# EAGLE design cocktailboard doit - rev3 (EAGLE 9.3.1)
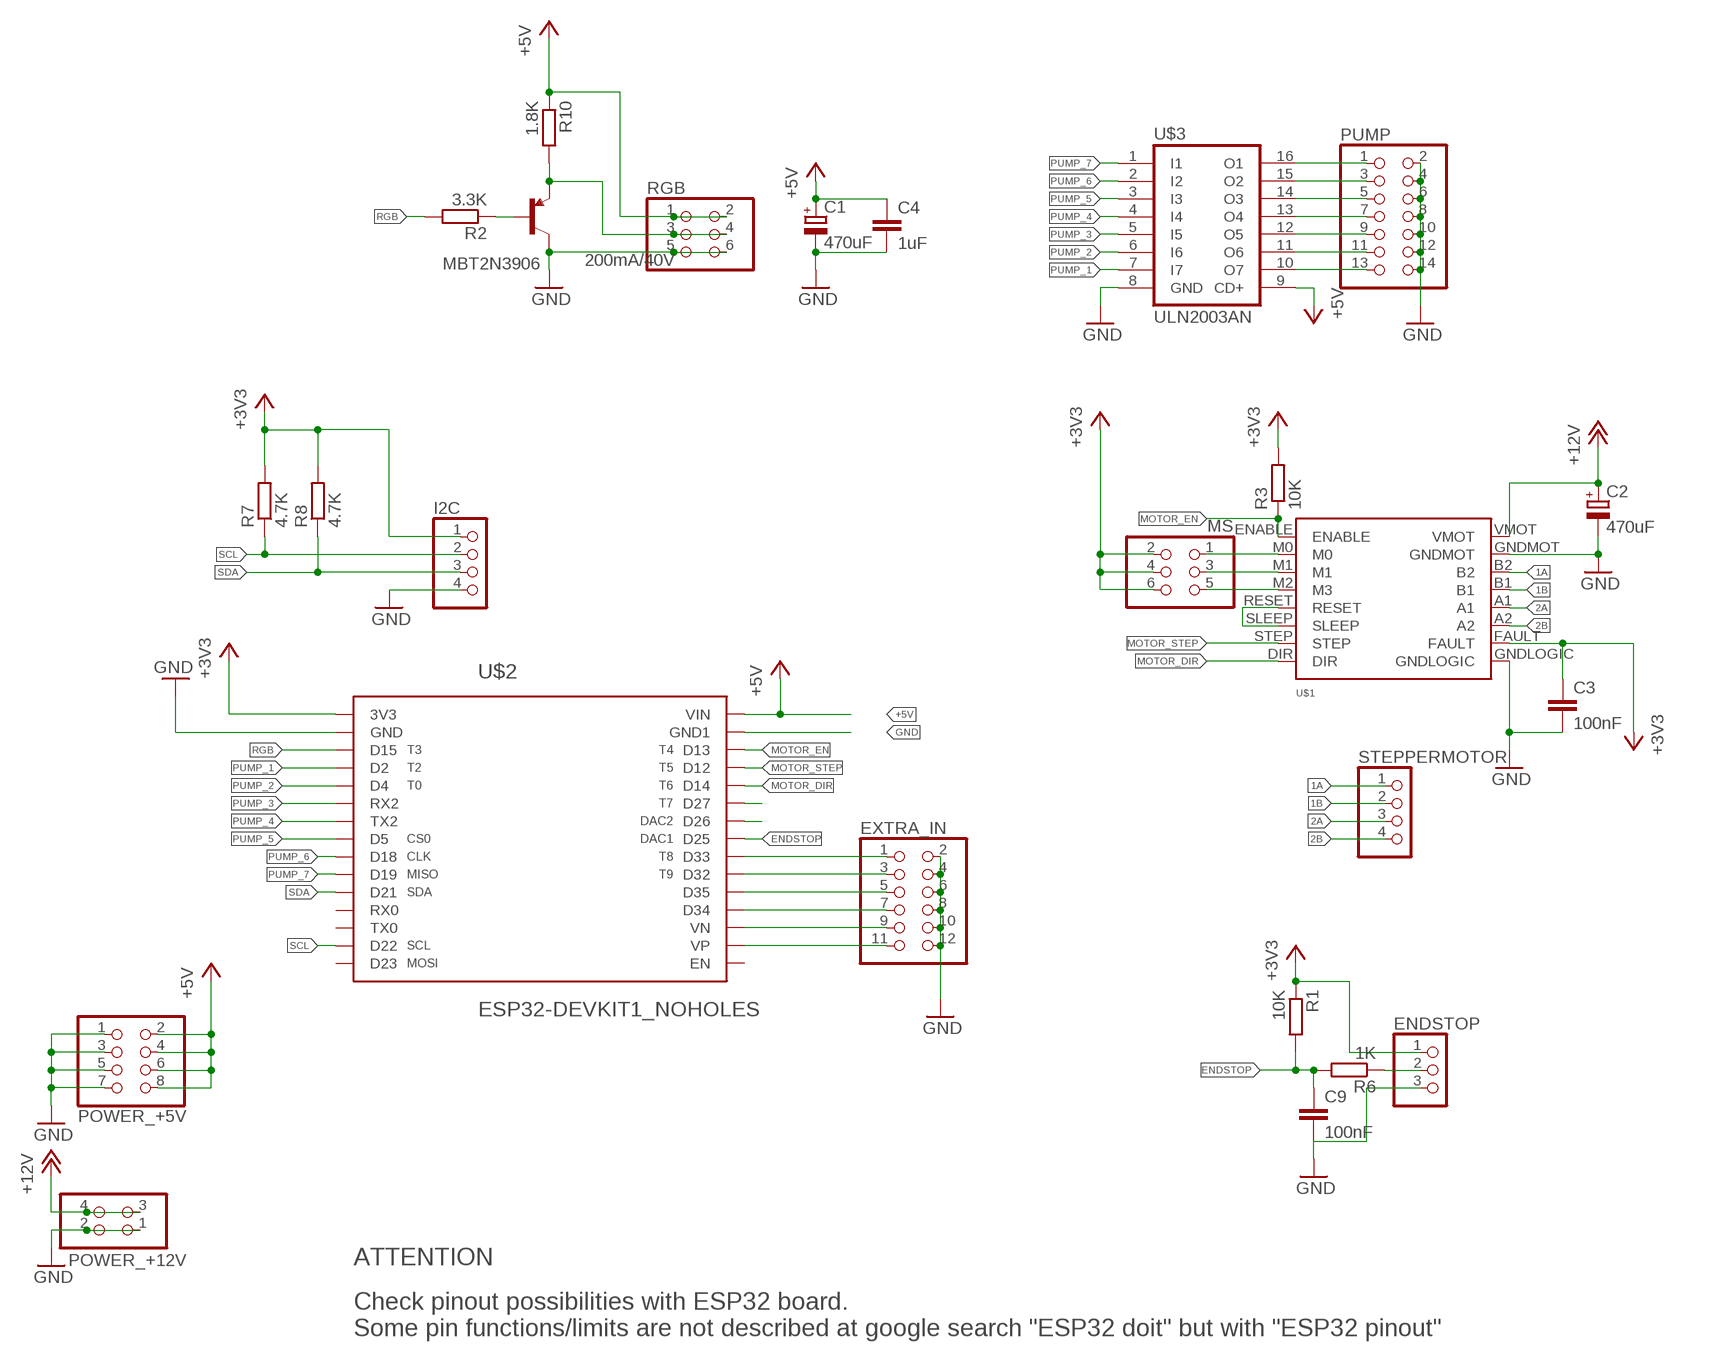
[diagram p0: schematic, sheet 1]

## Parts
C1  470uF  CPOL-EUE3.5-8  [E3,5-8]
C2  470uF  CPOL-EUE3.5-8  [E3,5-8]
C3  100nF  C-EUC1206  [C1206]
C4  1uF  C-EUC1206  [C1206]
C9  100nF  C-EUC1206  [C1206]
ENDSTOP  PINHD-1X3  [1X03]
EXTRA_IN  PINHD-2X6  [2X06]
I2C  PINHD-1X4  [1X04]
MBT2N3906  200mA/40V  TRANS_PNP-PMBT3906|MMBT3906L  [SOT23-3]
MS  PINHD-2X3  [2X03]
POWER_+5V  PINHD-2X4  [2X04]
POWER_+12V  PINHD-2X2  [2X02]
PUMP  PINHD-2X7  [2X07]
R1  10K  R-EU_R1206  [R1206]
R2  3.3K  R-EU_R1206  [R1206]
R3  10K  R-EU_R1206  [R1206]
R6  1K  R-EU_R1206  [R1206]
R7  4.7K  R-EU_R1206  [R1206]
R8  4.7K  R-EU_R1206  [R1206]
R10  1.8K  R-EU_R1206  [R1206]
RGB  PINHD-2X3  [2X03]
STEPPERMOTOR  PINHD-1X4  [1X04]
U$1  DRV8825  [DRV8825]
U$2  ESP32-DEVKIT1_NOHOLES  [NODELUA-ESP32DEVKIT1-NOHOLES]
U$3  ULN2003AN  [DIL16]

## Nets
1A: STEPPERMOTOR.1 U$1.B2
1B: STEPPERMOTOR.2 U$1.B1
2A: STEPPERMOTOR.3 U$1.A1
2B: STEPPERMOTOR.4 U$1.A2
+3V3: C3.1 ENDSTOP.1 I2C.1 MS.2 MS.4 MS.6 R1.1 R3.2 R7.2 R8.2 U$1.FAULT U$2.P$1(3V3)
+5V: C1.+ C4.1 POWER_+5V.2 POWER_+5V.4 POWER_+5V.6 POWER_+5V.8 R10.1 RGB.1 RGB.2 U$2.P$30(VIN) U$3.9(CD+)
+12V: C2.+ POWER_+12V.3 POWER_+12V.4 U$1.VMOT
ENDSTOP: C9.1 R1.2 R6.2 U$2.P$23(D25)
GND: C1.- C2.- C3.2 C4.2 C9.2 ENDSTOP.3 EXTRA_IN.2 EXTRA_IN.4 EXTRA_IN.6 EXTRA_IN.8 EXTRA_IN.10 EXTRA_IN.12 I2C.4 MBT2N3906.3(C) POWER_+5V.1 POWER_+5V.3 POWER_+5V.5 POWER_+5V.7 POWER_+12V.1 POWER_+12V.2 PUMP.2 PUMP.4 PUMP.6 PUMP.8 PUMP.10 PUMP.12 PUMP.14 RGB.5 RGB.6 U$1.GNDLOGIC U$1.GNDMOT U$2.P$2(GND) U$2.P$29(GND1) U$3.8(GND)
MOTOR_DIR: U$1.DIR U$2.P$26(D14)
MOTOR_EN: R3.1 U$1.ENABLE U$2.P$28(D13)
MOTOR_STEP: U$1.STEP U$2.P$27(D12)
N$1: MBT2N3906.1(B) R2.1
N$2: MS.1 U$1.M0
N$3: MS.3 U$1.M1
N$4: MS.5 U$1.M2(M3)
N$5: U$1.RESET U$1.SLEEP
N$6: ENDSTOP.2 R6.1
N$7: MBT2N3906.2(E) R10.2 RGB.3 RGB.4
N$8: PUMP.1 U$3.16(O1)
N$9: PUMP.3 U$3.15(O2)
N$10: PUMP.5 U$3.14(O3)
N$11: PUMP.7 U$3.13(O4)
N$12: PUMP.9 U$3.12(O5)
N$13: PUMP.11 U$3.11(O6)
N$14: PUMP.13 U$3.10(O7)
N$15: EXTRA_IN.1 U$2.P$22(D33)
N$16: EXTRA_IN.3 U$2.P$21(D32)
N$17: EXTRA_IN.5 U$2.P$20(D35)
N$18: U$2.P$25(D27)
N$19: U$2.P$24(D26)
N$20: EXTRA_IN.7 U$2.P$19(D34)
N$21: EXTRA_IN.9 U$2.P$18(VN)
N$22: EXTRA_IN.11 U$2.P$17(VP)
PUMP_1: U$2.P$4(D2) U$3.7(I7)
PUMP_2: U$2.P$5(D4) U$3.6(I6)
PUMP_3: U$2.P$6(RX2) U$3.5(I5)
PUMP_4: U$2.P$7(TX2) U$3.4(I4)
PUMP_5: U$2.P$8(D5) U$3.3(I3)
PUMP_6: U$2.P$9(D18) U$3.2(I2)
PUMP_7: U$2.P$10(D19) U$3.1(I1)
RGB: R2.2 U$2.P$3(D15)
SCL: I2C.2 R7.1 U$2.P$14(D22)
SDA: I2C.3 R8.1 U$2.P$11(D21)
Unconnected: U$2.P$12(RX0) U$2.P$13(TX0) U$2.P$15(D23) U$2.P$16(EN)

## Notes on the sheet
- ATTENTION
- Check pinout possibilities with ESP32 board.
  Some pin functions/limits are not described at google search "ESP32 doit" but with "ESP32 pinout"

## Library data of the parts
C1 C2 = resistor:CPOL-EU: POLARIZED CAPACITOR, European symbol
C3 C4 C9 = resistor:C-EU: CAPACITOR, European symbol
ENDSTOP = pinhead:PINHD-1X3: PIN HEADER
EXTRA_IN = pinhead:PINHD-2X6: PIN HEADER
I2C STEPPERMOTOR = pinhead:PINHD-1X4: PIN HEADER
MBT2N3906 = SparkFun-DiscreteSemi:TRANS_PNP: PNP transistor Current controlled devices typically used to amplify current or used as a switch. SparkFun Products: SparkFun Serial Enabled 16x2 LCD - Red on Black SparkFun Logomatic; PROD_ID: TRANS-08052
MS RGB = pinhead:PINHD-2X3: PIN HEADER
POWER_+5V = pinhead:PINHD-2X4: PIN HEADER
POWER_+12V = pinhead:PINHD-2X2: PIN HEADER
PUMP = pinhead:PINHD-2X7: PIN HEADER
R1 R3 R6 = resistor:R-EU_: RESISTOR, European symbol
R2 R7 R8 R10 = rcl:R-EU_: RESISTOR, European symbol; SPICEPREFIX: R
U$1 = stepper library:DRV8825
U$2 = ESP32 Doit DevKit 1:ESP32-DEVKIT1_NOHOLES; SPICEPREFIX: X
U$3 = uln-udn:ULN2003A: DRIVER ARRAY

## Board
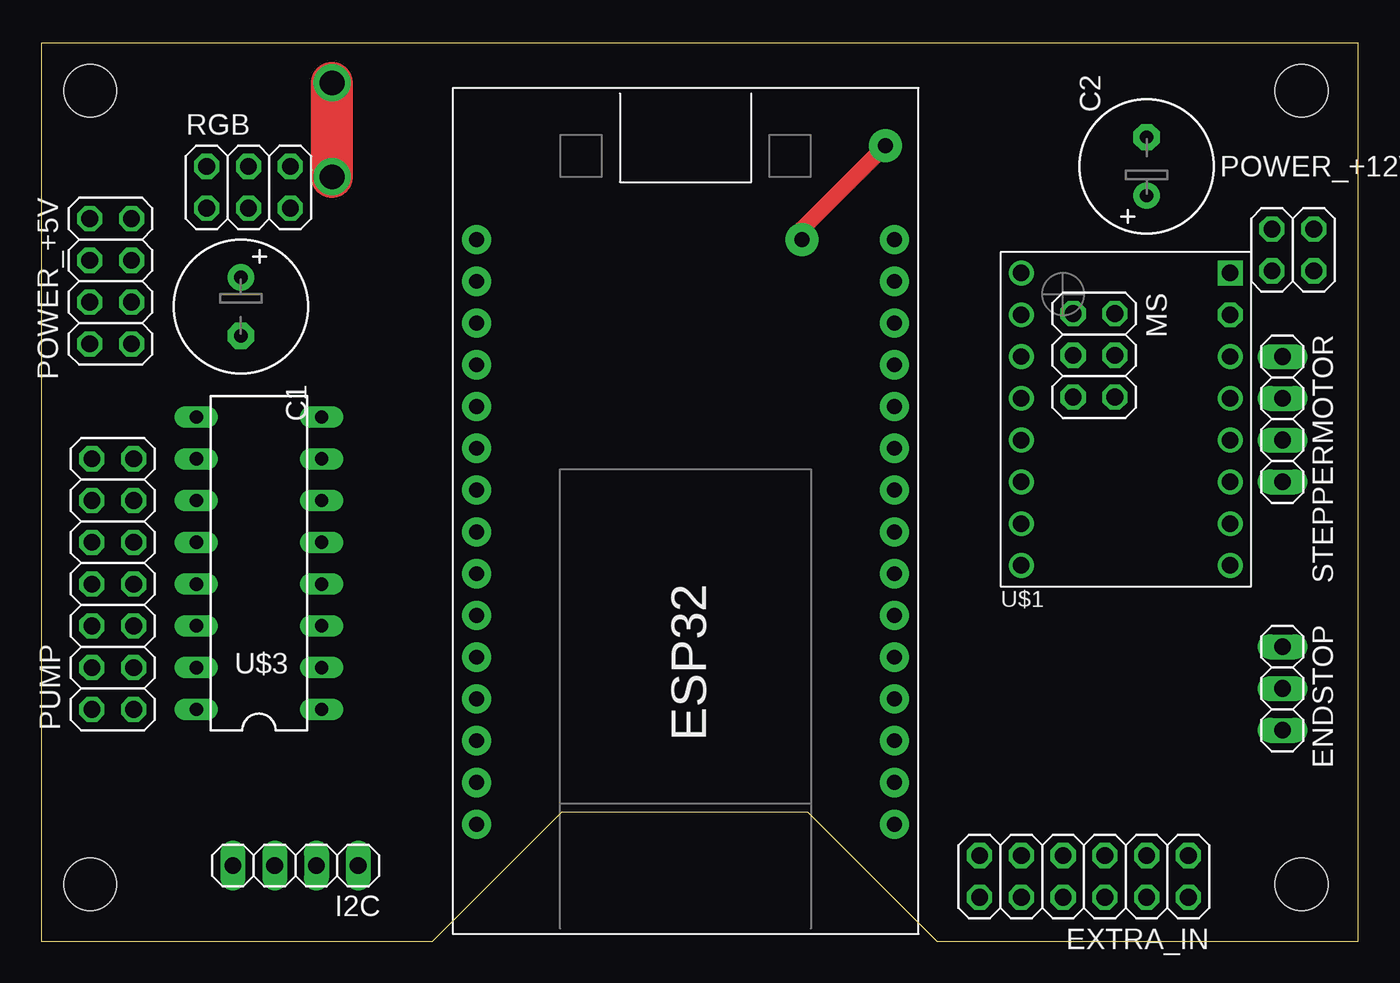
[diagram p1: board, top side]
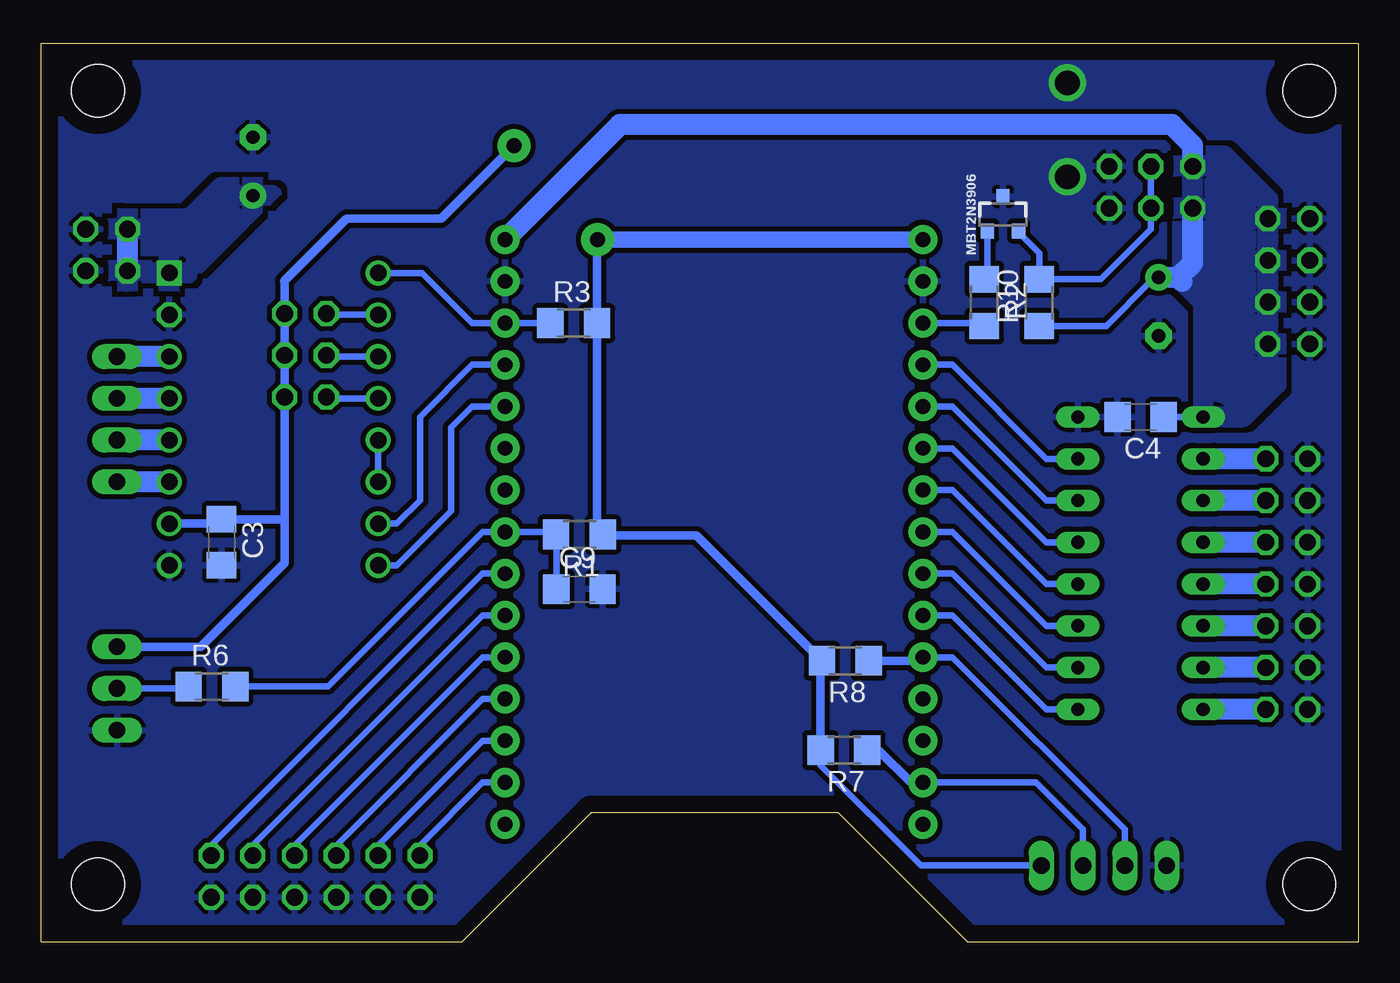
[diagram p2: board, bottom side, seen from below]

Size 80.09 x 54.63 mm. Coordinates in mm from the lower left corner, seen from the top.
Outline: 80.09,54.63 0,54.63 0,0 23.77,0 31.64,7.87 46.64,7.87 54.5,0 80.09,0 80.09,54.63
Copper layers (1*16): Top 0.035mm / dielectric 1.5mm / Bottom 0.035mm
Design rules "default": minimum track width 6mil, minimum drill 0.35mm, track to track 6mil, track to pad 6mil, pad to pad 6mil, via to via 6mil, smd to smd 6mil, copper to edge 40mil, drill to drill 6mil, minimum pad ring 10mil, minimum via ring 8mil, stop-mask expansion 4mil, vias tented up to drill 0mil, thermal gap 10mil
Holes 3.2 mm at 76.64,51.75 2.98,51.75 2.98,3.5 76.64,3.5

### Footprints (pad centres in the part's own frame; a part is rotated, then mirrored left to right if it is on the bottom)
E3,5-8 = drill 0.813 pad 1.6: + -1.778,0 | drill 0.813 pad 1.6 octagon: - 1.778,0
C1206 = smd 1.6 x 1.8: 1 -1.4,0; 2 1.4,0
1X03 = drill 1.016 long: 1 -2.54,0; 2 0,0; 3 2.54,0
2X06 = drill 1.016 octagon: 1 -6.35,-1.27; 2 -6.35,1.27; 3 -3.81,-1.27; 4 -3.81,1.27; 5 -1.27,-1.27; 6 -1.27,1.27; 7 1.27,-1.27; 8 1.27,1.27; 9 3.81,-1.27; 10 3.81,1.27; 11 6.35,-1.27; 12 6.35,1.27
1X04 = drill 1.016 long: 1 -3.81,0; 2 -1.27,0; 3 1.27,0; 4 3.81,0
SOT23-3 = smd 0.8 x 0.9: 1 -0.95,-1; 2 0.95,-1; 3 0,1.1
2X03 = drill 1.016 octagon: 1 -2.54,-1.27; 2 -2.54,1.27; 3 0,-1.27; 4 0,1.27; 5 2.54,-1.27; 6 2.54,1.27
2X04 = drill 1.016 octagon: 1 -3.81,-1.27; 2 -3.81,1.27; 3 -1.27,-1.27; 4 -1.27,1.27; 5 1.27,-1.27; 6 1.27,1.27; 7 3.81,-1.27; 8 3.81,1.27
2X02 = drill 1.016 octagon: 1 -1.27,-1.27; 2 -1.27,1.27; 3 1.27,-1.27; 4 1.27,1.27
2X07 = drill 1.016 octagon: 1 -7.62,-1.27; 2 -7.62,1.27; 3 -5.08,-1.27; 4 -5.08,1.27; 5 -2.54,-1.27; 6 -2.54,1.27; 7 0,-1.27; 8 0,1.27; 9 2.54,-1.27; 10 2.54,1.27; 11 5.08,-1.27; 12 5.08,1.27; 13 7.62,-1.27; 14 7.62,1.27
R1206 = smd 1.6 x 1.803: 1 -1.422,0; 2 1.422,0
DRV8825 = drill 1: A1 6.35,-11.43; A2 6.35,-13.97; B1 6.35,-8.89; B2 6.35,-6.35; DIR -6.35,-19.05; ENABLE -6.35,-1.27; FAULT 6.35,-16.51; GNDLOGIC 6.35,-19.05; M0 -6.35,-3.81; M1 -6.35,-6.35; M2 -6.35,-8.89; RESET -6.35,-11.43; SLEEP -6.35,-13.97; STEP -6.35,-16.51 | drill 1 octagon: GNDMOT 6.35,-3.81 | drill 1 square: VMOT 6.35,-1.27
NODELUA-ESP32DEVKIT1-NOHOLES = drill 0.9 pad 1.778: P$1 16.51,12.7; P$2 13.97,12.7; P$3 11.43,12.7; P$4 8.89,12.7; P$5 6.35,12.7; P$6 3.81,12.7; P$7 1.27,12.7; P$8 -1.27,12.7; P$9 -3.81,12.7; P$10 -6.35,12.7; P$11 -8.89,12.7; P$12 -11.43,12.7; P$13 -13.97,12.7; P$14 -16.51,12.7; P$15 -19.05,12.7; P$16 -19.05,-12.7; P$17 -16.51,-12.7; P$18 -13.97,-12.7; P$19 -11.43,-12.7; P$20 -8.89,-12.7; P$21 -6.35,-12.7; P$22 -3.81,-12.7; P$23 -1.27,-12.7; P$24 1.27,-12.7; P$25 3.81,-12.7; P$26 6.35,-12.7; P$27 8.89,-12.7; P$28 11.43,-12.7; P$29 13.97,-12.7; P$30 16.51,-12.7
DIL16 = drill 0.813 long: 1 -8.89,-3.81; 2 -6.35,-3.81; 3 -3.81,-3.81; 4 -1.27,-3.81; 5 1.27,-3.81; 6 3.81,-3.81; 7 6.35,-3.81; 8 8.89,-3.81; 9 8.89,3.81; 10 6.35,3.81; 11 3.81,3.81; 12 1.27,3.81; 13 -1.27,3.81; 14 -3.81,3.81; 15 -6.35,3.81; 16 -8.89,3.81

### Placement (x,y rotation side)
C1  12.14,38.62 270 top
C2  67.22,47.15 90 top
C3  69.12,24.29 270 bottom
C4  13.24,31.91 180 bottom
C9  47.36,21.44 0 bottom
ENDSTOP  75.48,15.4 270 top
EXTRA_IN  63.41,3.97 180 top
I2C  15.47,4.64 180 top
MBT2N3906  21.61,44.22 0 bottom
MS  64.02,35.66 270 top
POWER_+5V  4.23,40.16 270 top
POWER_+12V  76.11,42.07 180 top
PUMP  4.36,21.75 90 top
R1  47.36,24.76 180 bottom
R2  22.75,38.87 270 bottom
R3  47.71,37.62 0 bottom
R6  69.7,15.52 0 bottom
R7  31.28,11.65 180 bottom
R8  31.2,17.08 180 bottom
R10  19.41,38.87 90 bottom
RGB  12.61,45.88 0 top
STEPPERMOTOR  75.48,31.77 270 top
U$1  65.95,41.93 0 top
U$2  39.19,26.2 90 top
U$3  13.24,23.02 90 top

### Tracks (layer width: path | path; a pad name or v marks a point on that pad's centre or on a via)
1A
  Bottom 1.27: U$1.B2 STEPPERMOTOR.1
1B
  Bottom 1.27: U$1.B1 STEPPERMOTOR.2
2A
  Bottom 1.27: U$1.A1 STEPPERMOTOR.3
2B
  Bottom 1.27: U$1.A2 STEPPERMOTOR.4
+3V3  (via drill 0.9 pad 2)
  Top 1.016: v51.34,48.42 46.27,43.34 v46.27,42.7
  Bottom 0.406: I2C.1 26.61,4.64 32.7,10.73 R7.2
  Bottom 0.508: R7.2 32.7,17 R8.2 40.24,24.7 45.88,24.7 R1.1 46.1,24.92 46.27,24.92 46.29,24.95 R3.2 46.29,42.68 v46.27,42.7 | v51.34,48.42 55.79,43.98 61.51,43.98 65.31,40.16 65.29,40.14 MS.2 MS.4 MS.6 65.29,25.56 | C3.1 69,25.69 | C3.1 69.39,25.42 U$1.FAULT | 65.29,25.56 65.29,23.04 70.39,17.94 ENDSTOP.1 | C3.1 65.42,25.69 65.29,25.56
  Bottom 1.016: U$2.P$1 v46.27,42.7
+5V
  Bottom 0.406: U$3.9 C4.1 | C1.+ 12.38,40.16 12.61,40.16 15.33,37.44 R10.1
  Bottom 1.27: RGB.2 10.07,48.42 11.34,49.69 44.9,49.69 U$2.P$30 | C1.+ 10.94,40.4 | 10.94,40.4 10.71,40.16 | 10.94,40.4 10.07,41.28 RGB.1
  pour Bottom (isolate 0.61): 10.71,47.78 10.71,40.16 9.44,38.89 9.44,31.91 7.02,31.91 4.99,33.94 4.99,44.61 8.17,47.78
+12V
  Bottom 1.27: POWER_+12V.4 POWER_+12V.3
  pour Bottom (isolate 0.61): 66.59,45.24 71.67,40.16 74.84,40.16 75.48,40.16 75.48,43.98 71.03,43.98 69.12,45.88 65.95,45.88
ENDSTOP
  Bottom 0.406: R6.2 62.66,15.52 53.25,24.92 U$2.P$23 48.94,24.92 R1.2 48.76,24.74 C9.1
GND  (via drill 1.5)
  Top 2.54: v17.69,46.52 v17.69,52.23
  pour Bottom (isolate 0.305, rank 5): 89.45,-4.29 89.45,56.67 -4.54,56.67 -4.54,-4.29
MOTOR_DIR
  Bottom 0.406: U$1.DIR 58.47,22.88 55.16,26.2 55.16,31.27 53.89,32.55 U$2.P$26
MOTOR_EN
  Bottom 0.406: U$1.ENABLE 56.93,40.66 53.89,37.62 U$2.P$28 R3.1
MOTOR_STEP
  Bottom 0.406: U$1.STEP 58.47,25.42 57.06,26.83 57.06,31.91 53.89,35.09 U$2.P$27
N$1
  Bottom 0.406: MBT2N3906.1 22.56,40.48 R2.1
N$2
  Bottom 0.406: U$1.M0 62.68,38.12 MS.1
N$3
  Bottom 0.406: U$1.M1 62.68,35.59 MS.3
N$4
  Bottom 0.406: U$1.M2 62.68,33.05 MS.5
N$5
  Bottom 0.406: U$1.SLEEP U$1.RESET
N$6
  Bottom 0.406: ENDSTOP.2 71.25,15.4 R6.1
N$7
  Bottom 0.406: RGB.3 12.61,43.98 | RGB.4 RGB.3 | MBT2N3906.2 20.7,43.18 19.41,41.88 R10.2 15.66,40.29 12.61,43.34 RGB.3
N$8
  Bottom 1.27: PUMP.1 U$3.16
N$9
  Bottom 1.27: PUMP.3 U$3.15
N$10
  Bottom 1.27: PUMP.5 U$3.14
N$11
  Bottom 1.27: PUMP.7 U$3.13
N$12
  Bottom 1.27: PUMP.9 U$3.12
N$13
  Bottom 1.27: PUMP.11 U$3.11
N$14
  Bottom 1.27: PUMP.13 U$3.10
N$15
  Bottom 0.406: U$2.P$22 53.25,22.38 69.76,5.88 EXTRA_IN.1
N$16
  Bottom 0.406: EXTRA_IN.3 67.22,5.88 53.25,19.84 U$2.P$21
N$17
  Bottom 0.406: EXTRA_IN.5 64.68,5.88 53.25,17.3 U$2.P$20
N$20
  Bottom 0.406: EXTRA_IN.7 62.14,5.88 53.25,14.77 U$2.P$19
N$21
  Bottom 0.406: EXTRA_IN.9 59.6,5.88 53.25,12.22 U$2.P$18
N$22
  Bottom 0.406: EXTRA_IN.11 57.06,5.88 53.25,9.69 U$2.P$17
PUMP_1
  Bottom 0.406: U$2.P$4 24.68,35.09 18.96,29.37 U$3.7
PUMP_2
  Bottom 0.406: U$2.P$5 24.68,32.55 18.96,26.83 U$3.6
PUMP_3
  Bottom 0.406: U$2.P$6 24.68,30 18.96,24.29 U$3.5
PUMP_4
  Bottom 0.406: U$2.P$7 24.68,27.46 18.96,21.75 U$3.4
PUMP_5
  Bottom 0.406: U$2.P$8 24.68,24.92 18.96,19.21 U$3.3
PUMP_6
  Bottom 0.406: U$2.P$9 24.68,22.38 18.96,16.67 U$3.2
PUMP_7
  Bottom 0.406: U$3.1 18.96,14.13 24.68,19.84 U$2.P$10
RGB
  Bottom 0.406: U$2.P$3 22.93,37.62 R2.2
SCL
  Bottom 0.406: I2C.2 16.74,6.83 19.6,9.69 U$2.P$14
  Bottom 0.508: U$2.P$14 27.21,9.69 29.17,11.65 R7.1
SDA
  Bottom 0.406: I2C.3 14.2,6.83 24.68,17.3 U$2.P$11
  Bottom 0.508: U$2.P$11 26.71,17.08 R8.1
